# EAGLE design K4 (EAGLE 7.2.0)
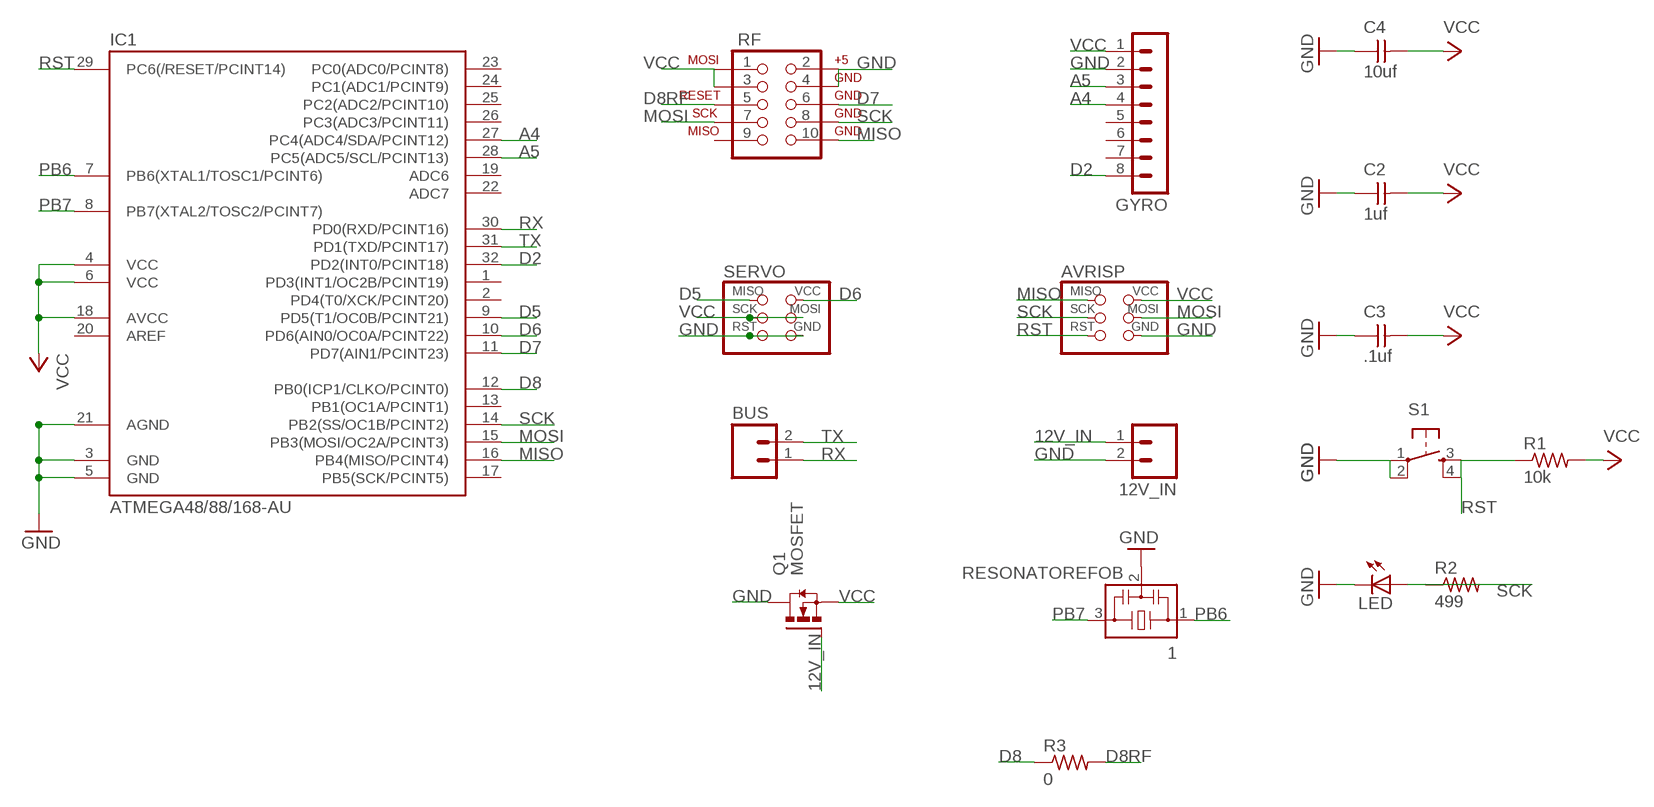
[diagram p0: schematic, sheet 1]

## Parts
1  RESONATOREFOB  [EFOBM]
12V_IN  M02  [1X02_LONGPADS]
AVRISP  AVRISPSMD  [2X03SMD]
BUS  M02  [1X02_LONGPADS]
C2  1uf  UNPOLARIZED_CAPACITOR1206  [1206]
C3  .1uf  UNPOLARIZED_CAPACITOR1206  [1206]
C4  10uf  UNPOLARIZED_CAPACITOR1206  [1206]
GYRO  MA08-1  [MA08-1]
IC1  ATMEGA48/88/168-AU  [TQFP32-08]
LED  LED1206  [1206]
Q1  MOSFET  N-HEXFET-2D_SOT232-  [SOT223]
R1  10k  RESISTOR1206  [1206]
R2  499  RESISTOR1206  [1206]
R3  0  RESISTOR1206  [1206]
RF  AVR_SPI_PROG  [AVR_ICSP]
S1  6MM_SWITCH6MM_SWITCH  [6MM_SWITCH]
SERVO  AVRISPSMD  [2X03SMD]

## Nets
12V_IN: 12V_IN.1 Q1.1(G)
A4: GYRO.4 IC1.27(PC4(ADC4/SDA/PCINT12))
A5: GYRO.3 IC1.28(PC5(ADC5/SCL/PCINT13))
D2: GYRO.8 IC1.32(PD2(INT0/PCINT18))
D5: IC1.9(PD5(T1/OC0B/PCINT21)) SERVO.1(MISO)
D6: IC1.10(PD6(AIN0/OC0A/PCINT22)) SERVO.2(VCC)
D7: IC1.11(PD7(AIN1/PCINT23)) RF.6
D8: IC1.12(PB0(ICP1/CLKO/PCINT0)) R3.1
D8RF: R3.2 RF.5
GND: 1.2 12V_IN.2 AVRISP.6(GND) C2.1 C3.1 C4.1 GYRO.2 IC1.3(GND) IC1.5(GND) IC1.21(AGND) LED.2(C) Q1.2(D) Q1.4(D) RF.2 RF.4 S1.1(P) S1.2(P1) SERVO.5(RST) SERVO.6(GND)
MISO: AVRISP.1(MISO) IC1.16(PB4(MISO/PCINT4)) RF.10
MOSI: AVRISP.4(MOSI) IC1.15(PB3(MOSI/OC2A/PCINT3)) RF.7
N$23: LED.1(A) R2.2
PB6: 1.1 IC1.7(PB6(XTAL1/TOSC1/PCINT6))
PB7: 1.3 IC1.8(PB7(XTAL2/TOSC2/PCINT7))
RST: AVRISP.5(RST) IC1.29(PC6(/RESET/PCINT14)) R1.1 S1.3(S) S1.4(S1)
RX: BUS.1 IC1.30(PD0(RXD/PCINT16))
SCK: AVRISP.3(SCK) IC1.14(PB2(SS/OC1B/PCINT2)) R2.1 RF.8
TX: BUS.2 IC1.31(PD1(TXD/PCINT17))
VCC: AVRISP.2(VCC) C2.2 C3.2 C4.2 GYRO.1 IC1.4(VCC) IC1.6(VCC) IC1.18(AVCC) Q1.3(S) R1.2 RF.1 RF.3 SERVO.3(SCK) SERVO.4(MOSI)
Unconnected: GYRO.5 GYRO.6 GYRO.7 IC1.1(PD3(INT1/OC2B/PCINT19)) IC1.2(PD4(T0/XCK/PCINT20)) IC1.13(PB1(OC1A/PCINT1)) IC1.17(PB5(SCK/PCINT5)) IC1.19(ADC6) IC1.20(AREF) IC1.22(ADC7) IC1.23(PC0(ADC0/PCINT8)) IC1.24(PC1(ADC1/PCINT9)) IC1.25(PC2(ADC2/PCINT10)) IC1.26(PC3(ADC3/PCINT11)) RF.9

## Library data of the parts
1 = fab:RESONATOR
12V_IN BUS = 01_SparkFun:M02: Header 2
AVRISP SERVO = 01_FAB_Hello:AVRISP
C2-C4 = ng:UNPOLARIZED_CAPACITOR: unpolarized_capacitor
GYRO = con-lstb:MA08-1: PIN HEADER
IC1 = atmega8:ATMEGA48/88/168
LED = ng:LED
Q1 = transistor-power:N-HEXFET-2D_?-*: HEXFET® Power MOSFET 2 Drain connects http://www.irf.com/product-info/datasheets/data/irll014n.pdf
R1-R3 = ng:RESISTOR
RF = 01_SparkFun:AVR_SPI_PROG: AVR ICSP Header This is the standard AVR In Circuit Serial Programming header. Minimal, but includes pin one indicator. Works with standard Olimex programmers. Also look for the 6-pin reduced version. Spark Fun Electronics SKU: PRT-00778
S1 = ng:6MM_SWITCH: OMRON SWITCH

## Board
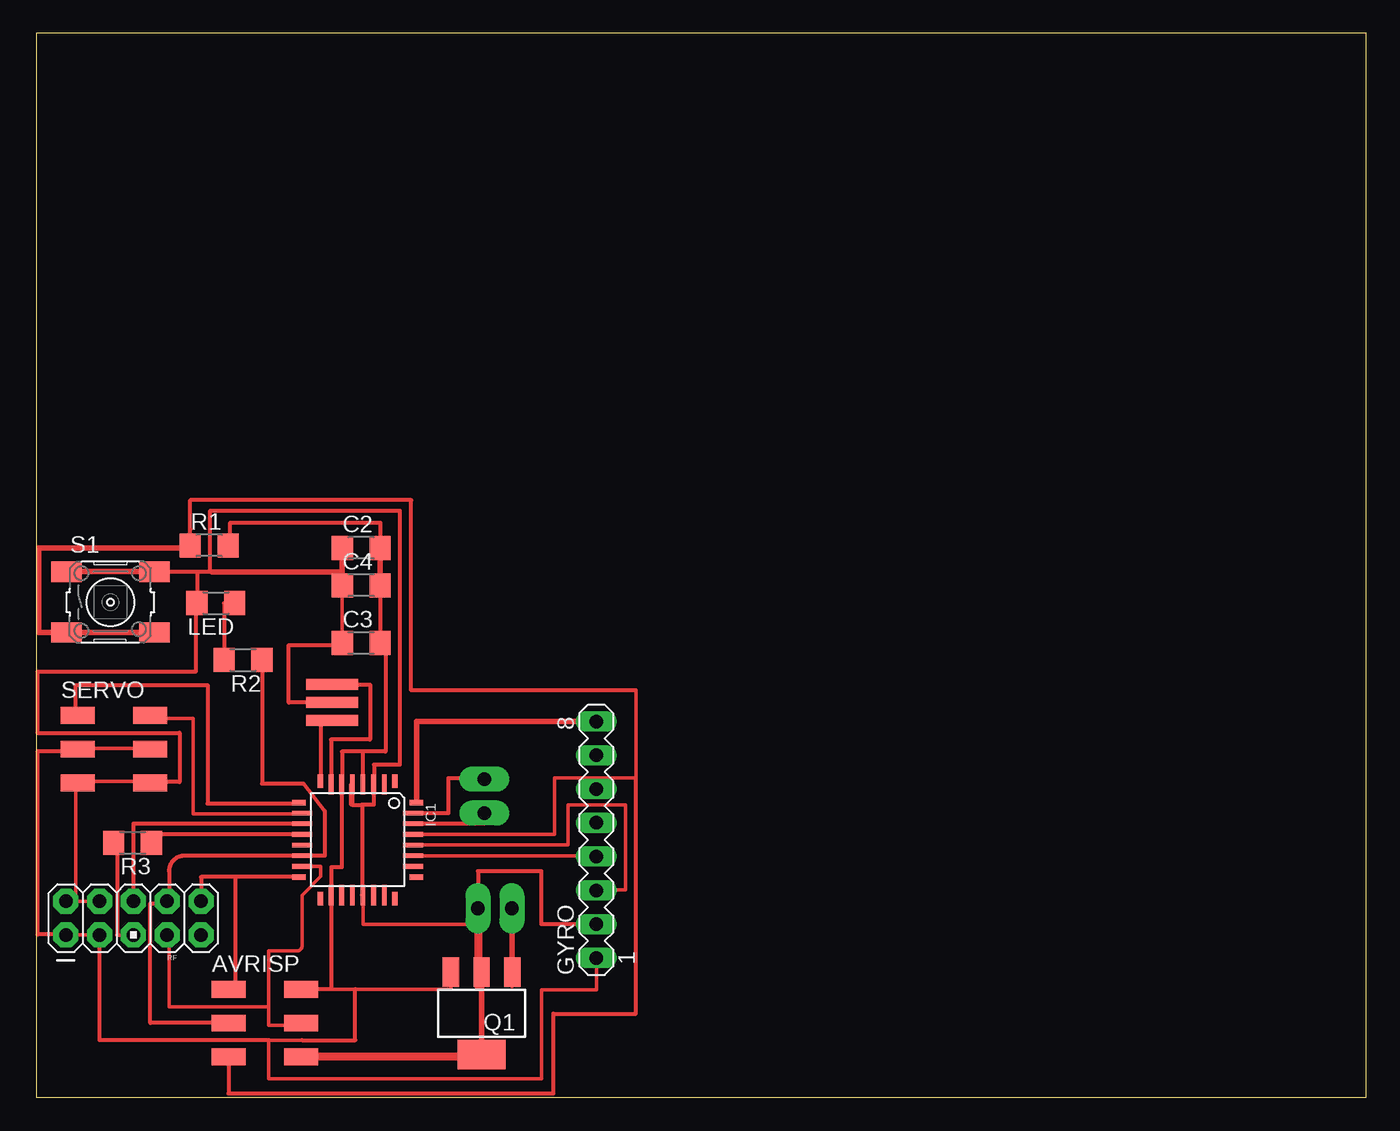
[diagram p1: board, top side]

Size 100 x 80 mm. Coordinates in mm from the lower left corner, seen from the top.
Outline: 0,0 100,0 100,80 0,80 0,0
Copper layers (1*16): Top 0.035mm / dielectric 1.5mm / Bottom 0.035mm
Design rules "default": minimum track width 10mil, minimum drill 24mil, track to track 8mil, track to pad 8mil, pad to pad 8mil, via to via 8mil, smd to smd 8mil, copper to edge 40mil, drill to drill 8mil, minimum pad ring 10mil, minimum via ring 8mil, stop-mask expansion 4mil, vias tented up to drill 0mil, thermal gap 10mil

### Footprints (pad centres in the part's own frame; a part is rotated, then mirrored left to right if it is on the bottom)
EFOBM = smd 0.8 x 3.9: 1 -1.35,0; 2 0,0; 3 1.35,0
1X02_LONGPADS = drill 1.016 pad 1.88 long: 1 0,0; 2 2.54,0
2X03SMD = smd 2.54 x 1.27: 1 -2.54,2.54; 2 2.92,2.54; 3 -2.54,0; 4 2.92,0; 5 -2.54,-2.54; 6 2.92,-2.54
1206 = smd 1.6 x 1.803: 1 -1.422,0; 2 1.422,0
MA08-1 = drill 1.016 long: 1 -8.89,0; 2 -6.35,0; 3 -3.81,0; 4 -1.27,0; 5 1.27,0; 6 3.81,0; 7 6.35,0; 8 8.89,0
TQFP32-08 = smd 1.016 x 0.406: 1 -4.42,2.8; 8 -4.42,-2.8; 17 4.42,-2.8; 24 4.42,2.8 | smd 1.524 x 0.356: 2 -4.166,2; 3 -4.166,1.2; 4 -4.166,0.4; 5 -4.166,-0.4; 6 -4.166,-1.2; 7 -4.166,-2; 18 4.166,-2; 19 4.166,-1.2; 20 4.166,-0.4; 21 4.166,0.4; 22 4.166,1.2; 23 4.166,2 | smd 0.406 x 1.016: 9 -2.8,-4.42; 16 2.8,-4.42; 25 2.8,4.42; 32 -2.8,4.42 | smd 0.356 x 1.524: 10 -2,-4.166; 11 -1.2,-4.166; 12 -0.4,-4.166; 13 0.4,-4.166; 14 1.2,-4.166; 15 2,-4.166; 26 2,4.166; 27 1.2,4.166; 28 0.4,4.166; 29 -0.4,4.166; 30 -1.2,4.166; 31 -2,4.166
SOT223 = smd 1.219 x 2.235: 1 -2.311,-3.099; 2 0,-3.099; 3 2.311,-3.099 | smd 3.6 x 2.2: 4 0,3.099
AVR_ICSP = drill 1.016 pad 1.88 octagon: 1 -1.27,5.08; 2 1.27,5.08; 3 -1.27,2.54; 4 1.27,2.54; 5 -1.27,0; 6 1.27,0; 7 -1.27,-2.54; 8 1.27,-2.54; 9 -1.27,-5.08; 10 1.27,-5.08
6MM_SWITCH = smd 2.286 x 1.524: 1 -3.302,2.286; 2 3.302,2.286; 3 -3.302,-2.286; 4 3.302,-2.286

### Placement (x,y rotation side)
1  22.27,29.69 270 top
12V_IN  35.77,14.21 180 top
AVRISP  17.02,5.59 0 top
BUS  33.69,21.37 90 top
C2  24.45,41.31 0 top
C3  24.45,34.15 0 top
C4  24.45,38.5 0 top
GYRO  42.12,19.37 90 top
IC1  24.18,19.37 270 top
LED  13.52,37.16 180 top
Q1  33.5,6.32 180 top
R1  13.02,41.5 0 top
R2  15.56,32.88 180 top
R3  7.26,19.14 180 top
RF  7.32,13.48 90 top
S1  5.59,37.23 0 top
SERVO  5.67,26.18 0 top

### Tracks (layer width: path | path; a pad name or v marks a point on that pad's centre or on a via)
12V_IN
  Top 0.406: 12V_IN.1 35.77,8.42 Q1.1
A4
  Top 0.254: IC1.27 42.12,18.17 GYRO.4
A5
  Top 0.254: IC1.28 40,18.97 40,22 44.3,22 44.3,15.6 42.12,15.6 GYRO.3
D2
  Top 0.406: IC1.32 28.6,28.26 GYRO.8
D5
  Top 0.305: SERVO.1 3,28.72 3,31 12.9,31 12.9,22.1 19.76,22.1 IC1.9
D6
  Top 0.254: IC1.10 20,21.3 11.8,21.3 11.8,28.5 7.75,28.5 SERVO.2
D7
  Top 0.305: IC1.11 7.32,20.57 RF.6
D8
  Top 0.305: IC1.12 8.68,19.77 R3.1
D8RF
  Top 0.305: R3.2 6.1,18.94 6.1,12.2 RF.5
GND
  Top 0.254: 3,14.75 RF.4 | IC1.21 24.58,13 33.23,13 | 3,23.75 7.5,23.75 7.96,23.7 SERVO.6 7.75,23.75 | 3,23.75 2.25,23.75 SERVO.5 | 3,14.75 3,23.75 | 3,14.75 RF.2 | 23,39.5 23,34.25 C3.1 | 11.5,36.75 LED.2
  Top 0.305: GYRO.2 38,13.02 38,17 33.23,17 12V_IN.2 | 13.25,39.5 13.1,39.5 | 13.1,39.5 13.1,39.52 | 13.1,39.52 13.1,44.1 27.35,44.1 27.35,25 25.4,25 25.4,23.54 IC1.3 25.38,22 24.5,22 | 7.96,23.7 10.8,23.7 10.8,27.4 0.1,27.4 0.1,32 12,32 12,36.75 11.5,36.75 | 1.2 19,29.69 19,34 23.03,34 C3.1 | 23.78,22 23.7,22 23.7,23.54 IC1.5 23.78,22 | 23.78,22 24.5,22 | 24.5,22 24.5,15.2 IC1.21 | 13.1,39.5 12.1,39.5 LED.2 | S1.2 13.1,39.52
  Top 0.406: C2.1 C4.1 23,39.5 13.25,39.5 | Q1.2 33.5,3.05 | S1.1 S1.2
  Top 0.61: 12V_IN.2 33.23,13 33.23,8.42 Q1.2 | Q1.4 33.5,3.05 AVRISP.6
MISO
  Top 0.305: IC1.16 15,16.57 | 15,16.57 12.4,16.57 RF.10 | AVRISP.1 15,8.13 15,16.57
MOSI
  Top 0.254: AVRISP.4 19.94,5.4 17.5,5.4 17.5,6.8 | 17.5,6.8 17.5,11 19.6,11 arc90 20,11.4 20,15.2 21.4,16.6 21.4,17.37 IC1.15 | 17.5,6.8 10,6.8 10,12 RF.7
N$23
  Top 0.305: LED.1 14.14,37.16 R2.2
PB6
  Top 0.305: 1.1 25.1,31.04 25.1,26.9 22.18,26.9 IC1.7
PB7
  Top 0.305: 1.3 21.38,28.34 IC1.8
RST
  Top 0.254: IC1.29 39,19.77 39,24 45.1,24 45.1,30.6
  Top 0.305: AVRISP.5 14.48,0.3 38.9,0.3 38.9,6.3 45.1,6.3 45.1,24 | 11.6,41.3 11.6,42.7 11.6,44.9 28.2,44.9 28.2,30.6 45.1,30.6
  Top 0.406: S1.3 S1.4 0.2,34.94 0.2,41.3 11.6,41.3 R1.1
RX
  Top 0.305: BUS.1 33.69,20.57 IC1.30
SCK
  Top 0.305: AVRISP.3 8.6,5.59 8.6,14.6 9.86,14.6 RF.8 arc90 10,14.89 10,17 arc-90 11.17,18.17 IC1.14 21.7,18.17 21.7,21.5 20.1,23.6 17,23.6 17,32.88 R2.1
TX
  Top 0.305: IC1.31 31,21.37 31,24 33.69,24 BUS.2
VCC
  Top 0.254: RF.3 RF.1 2,12.25 | GYRO.1 42.12,8.1 38,8.1 38,1.4 17.5,1.4 17.5,4.3 20,4.3 | Q1.3 31.19,8.13 24,8.13 21,8.13 AVRISP.2 | SERVO.4 7.5,26.25 2.25,26.25 SERVO.3 2,26 | 23,24.25 23,23.75 IC1.6
  Top 0.305: C4.2 C3.2 26.27,34.15 26.27,26 24.58,26 | R1.2 14.6,41.5 14.6,43.2 25.87,43.2 C2.2 | 2,26 0.1,26 0.1,12.25 2,12.25 | 24.58,26 23,26 23,23.54 IC1.6 22.98,17.3 22.2,17.3 22.2,15.2 IC1.18 22.18,8.13 21,8.13 | IC1.4 24.58,26 | 17.5,4.3 4.78,4.3 RF.3 | 20,4.3 24,4.3 24,8.13
  Top 0.406: C2.2 C4.2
